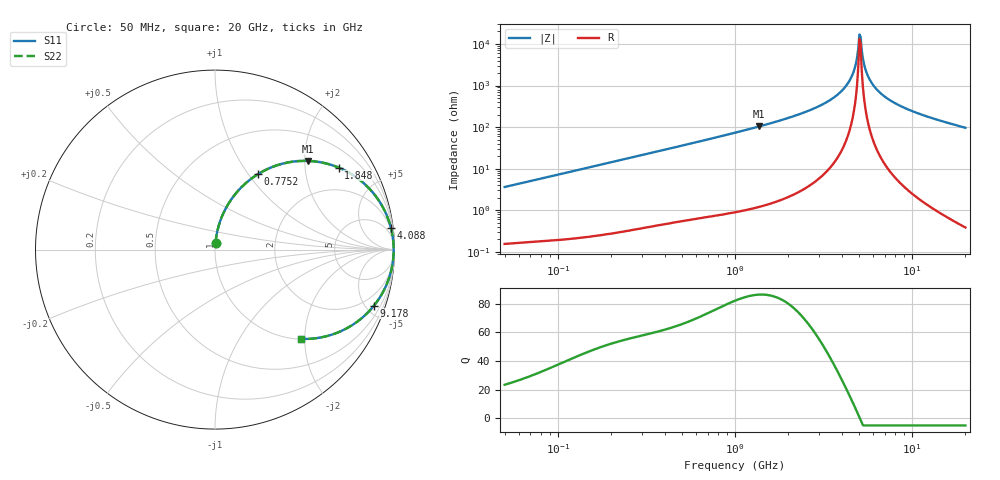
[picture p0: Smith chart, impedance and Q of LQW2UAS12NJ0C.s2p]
!Murata Part Number: LQW2UAS12NJ0C
!These Parameters are Measured in Series Mode Connection
!  o--[Z]--o
!Port1  Port2
!  o-------o
!Freq. Start=50[MHz] Stop=20[GHz], 401[Steps]
# Hz S RI R 50
!Freq.(Hz) S11(Real) S11(Imag) S21(Real) S21(Imag) S12(Real) S12(Imag) S22(Real) S22(Imag)
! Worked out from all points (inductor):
!   401 points, 50 MHz to 20 GHz, reference 50 ohm
!   read as one part in series: L = 11.4 nH near 51.52 MHz
!   highest Q = 86.5 at 1.37 GHz (marker M1), where L = 12 nH
!   self-resonance near 5.041 GHz
!   S11 on the Smith chart (normalised r, x): 50 MHz: 1.00, +0.07; 775.2 MHz: 1.01, +1.12; 1.848 GHz: 1.04, +2.99; 4.088 GHz: 2, +16; 9.178 GHz: 1.07, -5.66; 20 GHz: 1.01, -1.93
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5e7  0.00283 0.0359  0.9972 -0.0359  0.9972 -0.0359  0.00283 0.0359
1.364002e8  0.0115 0.0961  0.9885 -0.0961  0.9885 -0.0961  0.0115 0.0961
3.721004e8  0.0691 0.2455  0.9309 -0.2455  0.9309 -0.2455  0.0691 0.2455
7.751977e8  0.2407 0.421  0.7593 -0.421  0.7593 -0.421  0.2407 0.421
1e9  0.3501 0.471  0.6499 -0.471  0.6499 -0.471  0.3501 0.471
1.369645e9  0.5179 0.4939  0.4821 -0.4939  0.4821 -0.4939  0.5179 0.4939
1.848039e9  0.6886 0.4571  0.3114 -0.4571  0.3114 -0.4571  0.6886 0.4571
2.728004e9  0.8747 0.3232  0.1253 -0.3232  0.1253 -0.3232  0.8747 0.3232
3.466789e9  0.9495 0.2072  0.0505 -0.2072  0.0505 -0.2072  0.9495 0.2072
4.087748e9  0.9805 0.1195  0.0195 -0.1195  0.0195 -0.1195  0.9805 0.1195
4.608136e9  0.9924 0.0536  0.00762 -0.0536  0.00762 -0.0536  0.9924 0.0536
4.81993e9  0.9945 0.0286  0.00549 -0.0286  0.00549 -0.0286  0.9945 0.0286
4.966507e9  0.9952 0.012  0.00478 -0.012  0.00478 -0.012  0.9952 0.012
5.117541e9  0.9954 -0.00474  0.00462 0.00474  0.00462 0.00474  0.9954 -0.00474
5.194772e9  0.9952 -0.0131  0.00476 0.0131  0.00476 0.0131  0.9952 -0.0131
5.433528e9  0.994 -0.0381  0.006 0.0381  0.006 0.0381  0.994 -0.0381
5.769027e9  0.9904 -0.0713  0.00963 0.0713  0.00963 0.0713  0.9904 -0.0713
6.406762e9  0.9786 -0.1289  0.0214 0.1289  0.0214 0.1289  0.9786 -0.1289
7.442007e9  0.9498 -0.2087  0.0502 0.2087  0.0502 0.2087  0.9498 -0.2087
9.178299e9  0.8862 -0.3116  0.1138 0.3116  0.1138 0.3116  0.8862 -0.3116
1.375312e10  0.6964 -0.4566  0.3036 0.4566  0.3036 0.4566  0.6964 -0.4566
2e10  0.4819 -0.4977  0.5181 0.4977  0.5181 0.4977  0.4819 -0.4977
